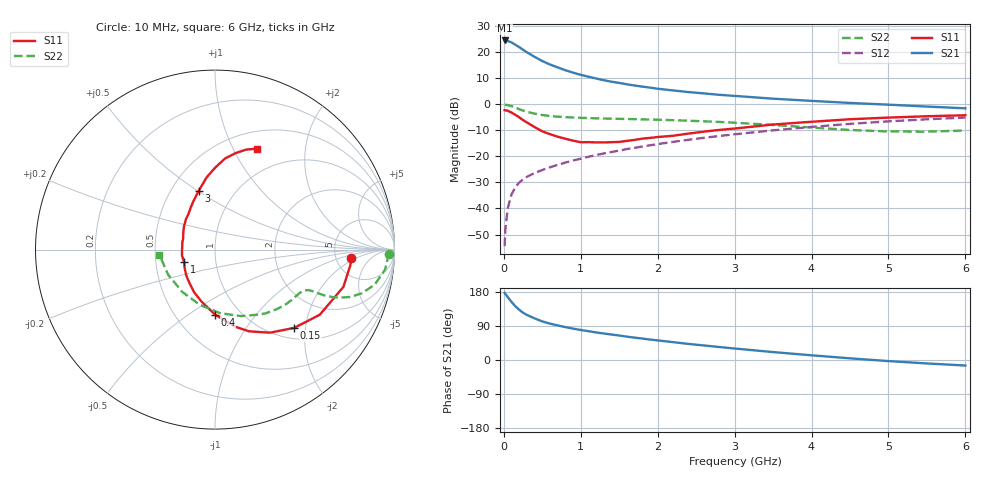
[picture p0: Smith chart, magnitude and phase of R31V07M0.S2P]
! SIEMENS Small Signal Semiconductors
! BFR181
! Si NPN RF Bipolar Junction Transistor in SOT23
! VCE = 1 V  IC = 7 mA
! Common Emitter S-Parameters:  May  1996
# GHz  S  MA  R  50
!  f  S11  S21  S12  S22
! GHz  MAG  ANG  MAG  ANG  MAG  ANG  MAG  ANG
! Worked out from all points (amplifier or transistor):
!   36 points, 10 MHz to 6 GHz, reference 50 ohm
!   highest |S21| = 24.3 dB at 10 MHz (marker M1)
!   |S21| within 3 dB of that: start of sweep to 222.4 MHz
!   unconditionally stable (mu >= 1): 663.3 MHz to 3.174 GHz
!   at 250 MHz: K = 0.58, MSG = 24.8 dB, |S12| = -28.8 dB
!   at 1.4 GHz: K = 1.15, MAG = 11.1 dB, |S12| = -18.4 dB
!   at 6 GHz: K = 0.92, MSG = 1.8 dB, |S12| = -5.2 dB
!   S11 on the Smith chart (normalised r, x): 10 MHz: 6.96, -1.57; 150 MHz: 1.23, -1.74; 400 MHz: 0.77, -0.64; 1 GHz: 0.70, -0.10; 3 GHz: 0.68, +0.50; 6 GHz: 0.70, +1.25
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0.01  0.7598 -3.6  16.48 177.2  0.0019 86.9  0.9719 -1.3
0.02  0.7593 -6.5  16.32 174.3  0.004 82.6  0.9639 -2.7
0.05  0.7451 -16.2  16.11 166.1  0.01 82.8  0.9547 -6.6
0.1  0.6873 -31.9  15.12 153.2  0.0186 74.8  0.9116 -12.3
0.15  0.6205 -44.6  13.65 141.7  0.0257 68.9  0.8526 -16.6
0.2  0.5557 -56.4  12.29 132.6  0.0314 66.5  0.798 -19.3
0.25  0.4936 -67.3  10.95 124.7  0.0362 63.1  0.747 -21.0
0.3  0.4432 -75.5  9.784 118.9  0.0404 63.0  0.7083 -22.0
0.4  0.362 -90.0  8 109.8  0.0479 61.9  0.6545 -22.8
0.5  0.3001 -104.3  6.643 101.8  0.0545 62.5  0.6153 -23.0
0.6  0.2646 -116.1  5.709 96.0  0.0614 62.8  0.5899 -23.1
0.8  0.2163 -137.5  4.441 86.8  0.0757 63.8  0.5612 -23.7
1  0.1853 -158.7  3.623 79.2  0.0899 65.3  0.5448 -24.9
1.1  0.1869 -169.5  3.334 76.0  0.0978 65.4  0.5385 -25.8
1.3  0.1835 174.8  2.854 69.9  0.1133 65.8  0.5282 -27.6
1.6  0.1971 153.9  2.384 61.6  0.1373 65.4  0.517 -31.2
2.2  0.2468 127.0  1.82 47.1  0.1884 62.8  0.4906 -40.1
3  0.3396 105.5  1.431 30.3  0.2634 56.9  0.4389 -55.5
3.5  0.4051 96.6  1.265 20.9  0.3134 52.1  0.3979 -68.6
4.5  0.5114 83.6  1.049 4.4  0.4172 40.2  0.3188 -105.5
5.5  0.5833 72.7  0.894 -9.1  0.5106 26.5  0.2963 -151.8
6  0.6098 67.4  0.828 -14.6  0.55 19.0  0.3107 -174.5
